(* Logix 5000 DataType export DriveStatus; software revision 20.01 *)

TYPE DriveStatus :
STRUCT
   Drive_Enable : BOOL;   // Drive Enable Input
   Drive_Homed : BOOL;   // Drive Home Input
   Drive_InMotion : BOOL;   // Drive In Motion Input
   Drive_EStop : BOOL;   // Drive E-Stop Input
   rsved_bit00 : BOOL;
   rsved_bit01 : BOOL;
   rsved_bit02 : BOOL;
   rsved_bit03 : BOOL;
   rsved_bit04 : BOOL;
   rsved_bit05 : BOOL;
   rsved_bit06 : BOOL;
   rsved_bit07 : BOOL;
   rsved_bit08 : BOOL;
   Drive_EthAvail : BOOL;   // Drive Ethernet Online
   rsved_bit09 : BOOL;
   rsved_bit10 : BOOL;
   rsved_bit11 : BOOL;
   rsved_bit12 : BOOL;
   rsved_bit13 : BOOL;
   rsved_bit14 : BOOL;
   Drive_BrakeOff : BOOL;   // Brake Output (0 - Enabled; 1- Not Enabled)
   rsved_bit15 : BOOL;
   rsved_bit16 : BOOL;
   rsved_bit17 : BOOL;
   rsrved_bit18 : BOOL;
   rsrved_bit19 : BOOL;
   rsrved_bit20 : BOOL;
   rsrved_bit21 : BOOL;
   rsrved_bit22 : BOOL;
   rsrved_bit23 : BOOL;
   rsrved_bit24 : BOOL;
   Drive_Control : BOOL;
END_STRUCT
END_TYPE
